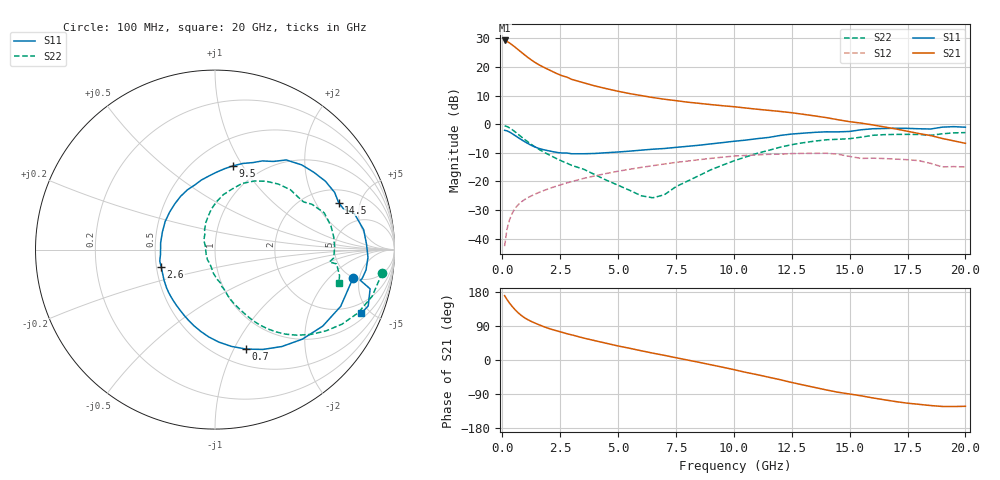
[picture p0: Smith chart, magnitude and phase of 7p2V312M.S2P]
! Infineon Technologies  Discrete & RF Semiconductors
! bfp620
! VCE =  2.3 V,  IC =  12 mA
! Common Emitter S-Parameters:  Sep 2002
# GHz  S  MA  R  50
!  f  S11  S21  S12  S22
! GHz  MAG  ANG  MAG  ANG  MAG  ANG  MAG  ANG
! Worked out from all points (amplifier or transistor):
!   59 points, 100 MHz to 20 GHz, reference 50 ohm
!   highest |S21| = 29.3 dB at 100 MHz (marker M1)
!   |S21| within 3 dB of that: start of sweep to 652.5 MHz
!   unconditionally stable (mu >= 1): 3.785 GHz to 10.55 GHz; 17.15 GHz to end of sweep
!   at 1 GHz: K = 0.56, MSG = 25.1 dB, |S12| = -26.1 dB
!   at 5.5 GHz: K = 1.05, MAG = 11.9 dB, |S12| = -15.7 dB
!   at 20 GHz: K = 1.29, MAG = 0.9 dB, |S12| = -14.9 dB
!   S11 on the Smith chart (normalised r, x): 100 MHz: 4.94, -4.04; 700 MHz: 0.67, -1.12; 2.6 GHz: 0.53, -0.11; 9.5 GHz: 0.75, +0.91; 14.5 GHz: 2.76, +3.17; 20 GHz: 1.31, -4.44
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0.1  0.7857 -11.5  29.22 169.9  0.0074 63.4  0.9408 -7.9
0.2  0.7683 -24.3  28.11 159.9  0.0144 68.9  0.9137 -16.5
0.3  0.7362 -35.4  26.62 151.2  0.0207 67.4  0.8714 -23.9
0.4  0.697 -45.7  24.93 143.4  0.0263 64.7  0.8206 -30.4
0.5  0.6561 -55.4  23.2 136.2  0.0314 62.0  0.7667 -36.2
0.6  0.6168 -64.4  21.53 129.7  0.0358 59.6  0.7132 -41.5
0.7  0.5804 -72.7  19.95 123.8  0.0397 57.5  0.662 -46.1
0.8  0.5469 -80.4  18.49 118.6  0.0433 55.7  0.6142 -50.1
1  0.4882 -94.0  15.92 110.0  0.0493 53.0  0.53 -56.4
1.2  0.4399 -105.5  13.82 103.3  0.0546 51.1  0.4611 -61.0
1.4  0.4029 -115.7  12.17 97.7  0.0597 49.7  0.4058 -64.4
1.9  0.351 -137.7  9.444 85.5  0.0721 47.3  0.31 -71.3
2.6  0.3147 -162.5  7.02 72.8  0.0896 43.8  0.2249 -77.3
3.5  0.3052 172.8  5.337 58.1  0.1129 38.2  0.1649 -86.1
5  0.3278 140.5  3.78 37.1  0.1511 27.0  0.086 -109.0
7  0.3775 107.3  2.743 12.3  0.2021 10.3  0.0586 158.2
9.5  0.478 77.7  2.114 -18.8  0.266 -14.4  0.1921 101.1
10.5  0.5281 66.6  1.928 -32.4  0.2856 -26.6  0.2675 88.0
13.5  0.7234 31.8  1.399 -72.5  0.3101 -60.7  0.5081 45.9
14.5  0.7371 20.8  1.201 -85.1  0.3003 -75.7  0.5471 32.5
17  0.8534 -2.9  0.829 -109.8  0.2463 -92.2  0.6655 5.9
20  0.8889 -23.5  0.465 -122.2  0.1791 -103.1  0.7148 -15.1
